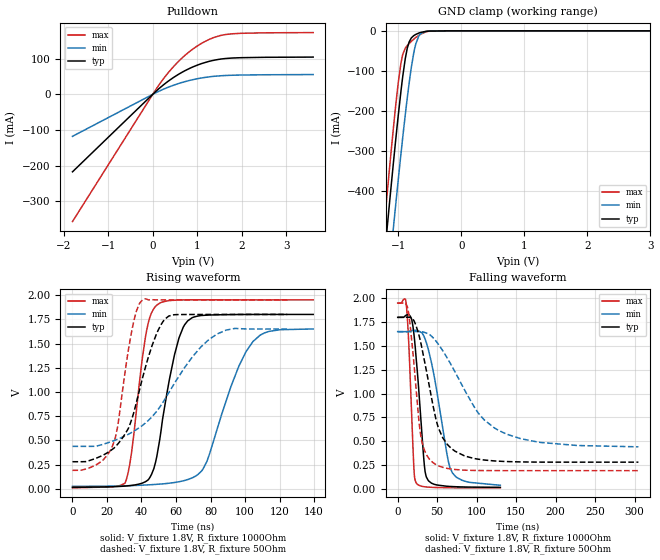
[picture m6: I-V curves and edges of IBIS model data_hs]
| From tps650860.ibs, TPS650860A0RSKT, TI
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|   data_hs Model
[Model]   data_hs
Model_type   I/O_open_drain
Polarity   Inverting
Vinl = 0.4
Vinh = 1.2
Vmeas = 0.9
Vref = 1.8
Cref = 50pF
Rref = 1000
|   typ   min   max
|   (nom PVT)   (fast PVT)   (slow PVT)
C_comp   1.676e-12   1.451e-12   1.832e-12
| Where nom  PVT is Nominal Process, 1.8V, 27C
|   Fast PVT is Strong Process,  1.95V, -40C
|   Slow PVT is Weak Process,   1.65V, 125C
[Voltage Range]   1.8   1.65   1.95
|Junction Temperature
[Temperature Range]   27   125   -40
[Pullup Reference]   1.8   1.65   1.95
[Pulldown Reference]   0   0   0
[Power Clamp Reference]   1.8   1.65   1.95
[GND Clamp Reference]   0   0   0
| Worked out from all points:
|   slope of the pulldown table from 0 to 0.27 V, typ, clamps not added: 9.17 ohm
|   GND clamp passes 1 mA (typ) near -0.54 V on its own axis
|   falling waveform, V_fixture 1.8V, R_fixture 1000Ohm: 20-80 % time 9.84ns typ, 19.8ns min, 5.71ns max; typ from 1.8 V to 0.015 V
|   rising waveform, V_fixture 1.8V, R_fixture 1000Ohm: 20-80 % time 10.8ns typ, 18.8ns min, 7.84ns max; typ from 0.015 V to 1.8 V
|   falling waveform, V_fixture 1.8V, R_fixture 50Ohm: 20-80 % time 24.2ns typ, 55.6ns min, 12.3ns max; typ from 1.8 V to 0.28 V
|   rising waveform, V_fixture 1.8V, R_fixture 50Ohm: 20-80 % time 15.4ns typ, 29.3ns min, 9.01ns max; typ from 0.28 V to 1.8 V
[Pulldown]
|   Voltage   I(typ)   I(min)   I(max)
-1.8V     -217.2mA   -117.7mA   -356.6mA
117mV     13.52mA    7.322mA    22.21mA
321.9mV   34.46mA    18.63mA    56.63mA
467.8mV   47.38mA    25.58mA    77.92mA
684mV     63.67mA    34.26mA    104.9mA
826.2mV   72.65mA    38.98mA    120mA
1.081V    85.55mA    45.61mA    141.9mA
1.263V    92.42mA    49mA       153.8mA
1.398V    96.23mA    50.82mA    160.5mA
1.642V    100.5mA    52.87mA    167.8mA
1.981V    102.8mA    54.13mA    171.1mA
3.6V      104.4mA    55.46mA    173.2mA
[GND Clamp]
|   Voltage   I(typ)   I(min)   I(max)
-1.8V     -1.585A    -1.712A    -1.529A
-1.417V   -903.9mA   -1.052A    -830.1mA
-1.201V   -532.4mA   -690.5mA   -448.4mA
-1.17V    -480.2mA   -639.5mA   -395mA
-1.076V   -327.4mA   -488.9mA   -240.6mA
-959.6mV  -153.1mA   -309.5mA   -82.58mA
-887.4mV  -67.95mA   -206.8mA   -42.91mA
-828mV    -27.88mA   -130.5mA   -31.56mA
-722.6mV  -8.948mA   -32.89mA   -16.64mA
-648.3mV  -4.138mA   -7.502mA   -8.538mA
-516.9mV  -657.9uA   -778.2uA   -1.114mA
3.6V      0A         0A         0A
[POWER Clamp]
|   Voltage   I(typ)   I(min)   I(max)
-1.8V     0A         0A         0A
0V        0A         0A         0A
3.6V      0A         0A         0A
[Ramp]
R_load = 1000
|   typ   min   max
dV/dt_r   1.07107/1.06427e-08   0.974924/1.86711e-08   1.1641/7.82039e-09
dV/dt_f   1.07107/9.83065e-09   0.974924/1.99465e-08   1.1641/5.70367e-09
[Falling Waveform]
V_fixture = 1.8V
V_fixture_min = 1.65V
V_fixture_max = 1.95V
R_fixture = 1000Ohm
|   Time   V(typ)   V(min)   V(max)
0s        1.8V       1.65V      1.95V
11.32ns   1.825V     1.65V      1.895V
14.03ns   1.828V     1.651V     1.524V
20.44ns   1.632V     1.663V     225.4mV
23.38ns   1.37V      1.663V     63.17mV
33.8ns    242mV      1.59V      21.35mV
38.65ns   87.22mV    1.467V     17.52mV
64.09ns   25.6mV     288.4mV    11.07mV
69.37ns   23.08mV    165.1mV    10.69mV
130ns     15.41mV    37.66mV    9.836mV
[Rising Waveform]
V_fixture = 1.8V
V_fixture_min = 1.65V
V_fixture_max = 1.95V
R_fixture = 1000Ohm
|   Time   V(typ)   V(min)   V(max)
0s        14.87mV    25.09mV    9.826mV
30.51ns   28.08mV    31mV       58.9mV
34.27ns   34.86mV    33.13mV    377.7mV
42.17ns   71.95mV    38.89mV    1.554V
48.87ns   333.3mV    46.26mV    1.896V
59.11ns   1.382V     64.86mV    1.946V
66.78ns   1.734V     95.05mV    1.951V
77.94ns   1.793V     283.6mV    1.951V
104.6ns   1.8V       1.521V     1.95V
139.5ns   1.8V       1.65V      1.95V
[Falling Waveform]
V_fixture = 1.8V
V_fixture_min = 1.65V
V_fixture_max = 1.95V
R_fixture = 50Ohm
|   Time   V(typ)   V(min)   V(max)
0s        1.8V       1.65V      1.95V
12.77ns   1.801V     1.65V      1.894V
20.85ns   1.76V      1.651V     1.286V
29.56ns   1.521V     1.649V     539.5mV
44.83ns   869mV      1.586V     274mV
52ns      629.6mV    1.512V     239.8mV
67.99ns   423.3mV    1.297V     207.1mV
101.9ns   310.9mV    795.7mV    191.9mV
127.6ns   289.8mV    613.8mV    190.7mV
304.8ns   279.5mV    440.6mV    190.5mV
[Rising Waveform]
V_fixture = 1.8V
V_fixture_min = 1.65V
V_fixture_max = 1.95V
R_fixture = 50Ohm
|   Time   V(typ)   V(min)   V(max)
0s        279.5mV    438.2mV    190.5mV
13.71ns   315.4mV    439.6mV    246.7mV
22.54ns   399.8mV    487.4mV    412.2mV
26.04ns   457.5mV    511mV      629.8mV
34.57ns   730.5mV    584.6mV    1.65V
40.78ns   1.156V     657mV      1.951V
48.55ns   1.592V     794.1mV    1.95V
55.85ns   1.784V     992.4mV    1.95V
83.82ns   1.8V       1.598V     1.95V
124.5ns   1.8V       1.65V      1.95V
